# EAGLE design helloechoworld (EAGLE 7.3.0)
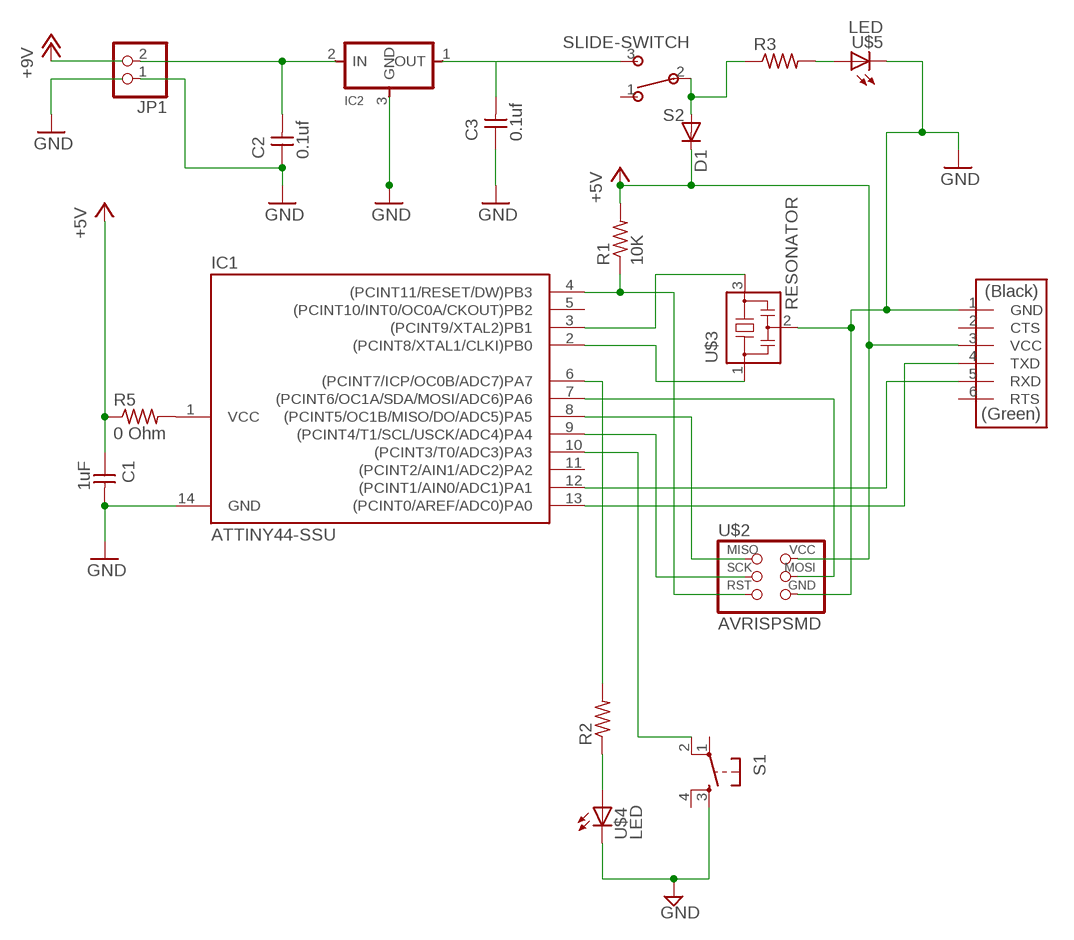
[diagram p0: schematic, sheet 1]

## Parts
C1  1uF  CAP-UNPOLARIZED  [C1206]
C2  0.1uf  CAP-UNPOLARIZED  [C1206]
C3  0.1uf  CAP-UNPOLARIZED  [C1206]
D1  DIODESOD123  [SOD123]
IC1  ATTINY44-SSU  [SOIC14]
IC2  REGULATORSOT23  [SOT23]
JP1  PINHD-1X2  [1X02]
R1  10K  RES-US1206  [R1206]
R2  RES-US1206  [R1206]
R3  RES-US1206  [R1206]
R5  0 Ohm  RES-US1206FAB  [R1206FAB]
S1  6MM_SWITCH6MM_SWITCH  [6MM_SWITCH]
S2  SLIDE-SWITCH  [AYZ0102AGRLC]
U$1  FTDI-SMD-HEADER  [1X06SMD]
U$2  AVRISPSMD  [2X03SMD]
U$3  RESONATOR  [EFOBM]
U$4  LED  [LED1206]
U$5  LED  [LED1206]

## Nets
+5V: C1.1 D1.CATHODE(C) R1.2 R5.1 U$1.3(VCC) U$2.2(VCC)
GND: C1.2 C2.1 C3.1 IC1.14(GND) IC2.3(GND) JP1.1 S1.3(S) U$1.1(GND) U$2.6(GND) U$3.2 U$4.2(C) U$5.2(C)
N$1: IC1.2((PCINT8/XTAL1/CLKI)PB0) U$3.1
N$2: IC1.8((PCINT5/OC1B/MISO/DO/ADC5)PA5) U$2.1(MISO)
N$3: IC1.3((PCINT9/XTAL2)PB1) U$3.3
N$4: IC1.6((PCINT7/ICP/OC0B/ADC7)PA7) R2.2
N$5: IC1.4((PCINT11/RESET/DW)PB3) R1.1 U$2.5(RST)
N$6: IC1.9((PCINT4/T1/SCL/USCK/ADC4)PA4) U$2.3(SCK)
N$7: IC1.7((PCINT6/OC1A/SDA/MOSI/ADC6)PA6) U$2.4(MOSI)
N$8: IC1.12((PCINT1/AIN0/ADC1)PA1) U$1.5(RXD)
N$9: IC1.13((PCINT0/AREF/ADC0)PA0) U$1.4(TXD)
N$10: R2.1 U$4.1(A)
N$11: IC1.10((PCINT3/T0/ADC3)PA3) S1.2(P1)
N$12: C2.2 IC2.2(IN) JP1.2
N$13: C3.2 IC2.1(OUT) S2.3
N$14: IC1.1(VCC) R5.2
N$16: D1.ANODE(A) R3.1 S2.2
N$17: R3.2 U$5.1(A)
Unconnected: IC1.5((PCINT10/INT0/OC0A/CKOUT)PB2) IC1.11((PCINT2/AIN1/ADC2)PA2) S1.1(P) S1.4(S1) S2.1 U$1.2(CTS) U$1.6(RTS)

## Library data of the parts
C1-C3 = fab:CAP-UNPOLARIZED
D1 = fab:DIODE: DIODE
IC1 = fab:ATTINY44
IC2 = fab:REGULATOR
JP1 = pinhead:PINHD-1X2: PIN HEADER
R1-R3 R5 = fab:RES-US: Resistor (US Symbol)
S1 = fab:6MM_SWITCH: OMRON SWITCH
S2 = fab:SLIDE-SWITCH: SMD slide-switch AYZ0102AGRLC as found in the fablab inventory. Includes the mounting holes. Made by Zaerc.
U$1 = fab:FTDI-SMD-HEADER
U$2 = fab:AVRISP
U$3 = fab:RESONATOR
U$4 U$5 = fab:LED: LED

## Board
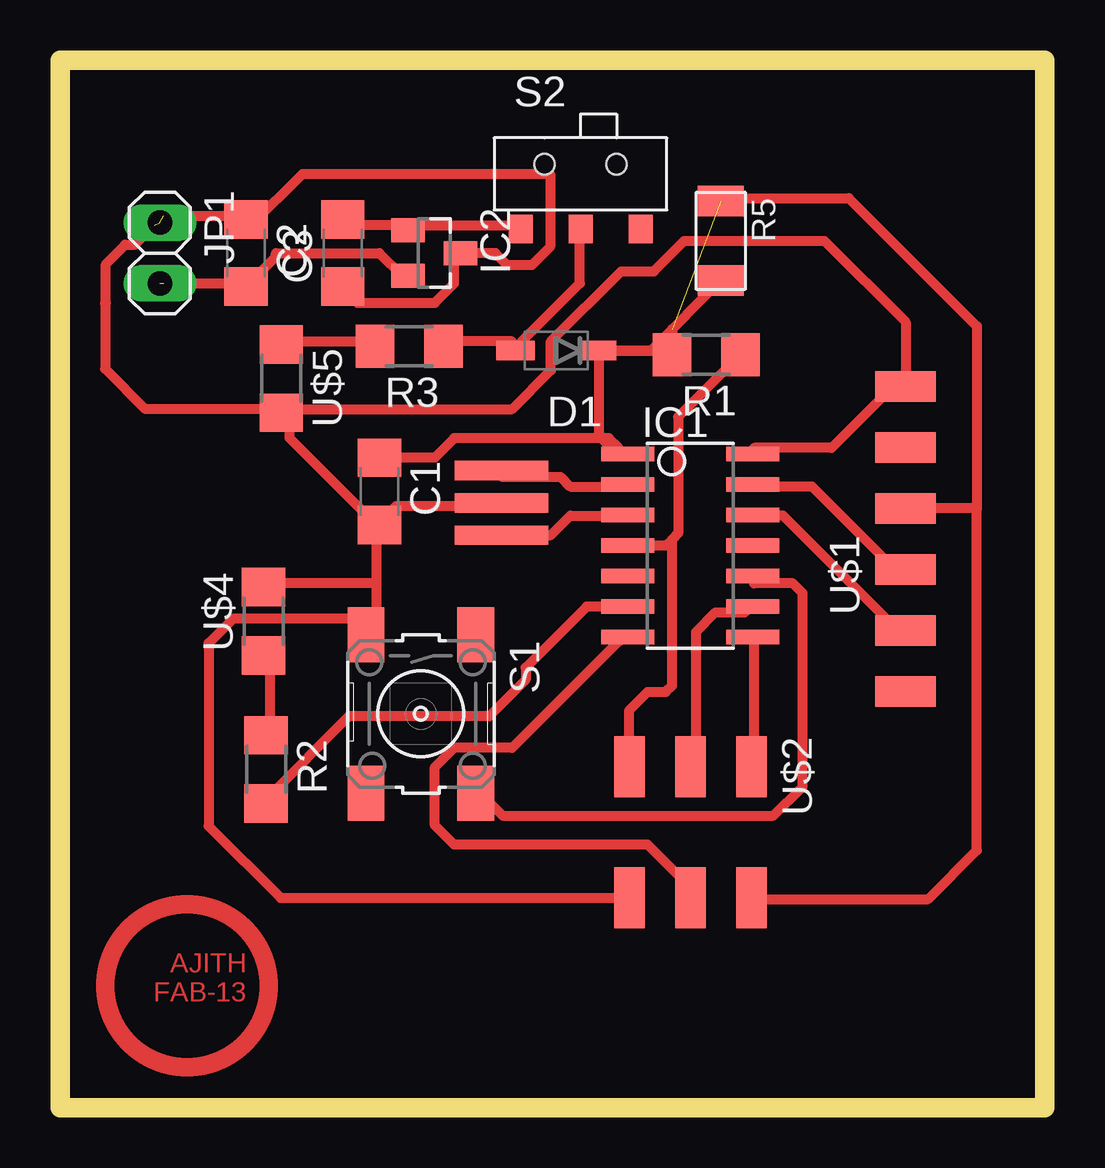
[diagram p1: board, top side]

Size 41.02 x 43.65 mm. Coordinates in mm from the lower left corner, seen from the top.
Outline: 0,0 41.02,0 41.02,43.65 0,43.65 0,0
Copper layers (1*16): Top 0.035mm / dielectric 1.5mm / Bottom 0.035mm
Design rules "default *": minimum track width 16mil, minimum drill 24mil, track to track 0.4mm, track to pad 0.4mm, pad to pad 0.4mm, via to via 0.4mm, smd to smd 0.4mm, copper to edge 40mil, drill to drill 16mil, minimum pad ring 10mil, minimum via ring 8mil, stop-mask expansion 4mil, vias tented up to drill 0mil, thermal gap 10mil

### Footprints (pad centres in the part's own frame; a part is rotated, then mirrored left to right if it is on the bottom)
C1206 = smd 1.6 x 1.8: 1 -1.4,0; 2 1.4,0
SOD123 = smd 1.6 x 0.8: ANODE 1.7,0; CATHODE -1.7,0
SOIC14 = smd 0.61 x 2.21: 1 -3.81,-2.603; 2 -2.54,-2.603; 3 -1.27,-2.603; 4 0,-2.603; 5 1.27,-2.603; 6 2.54,-2.603; 7 3.81,-2.603; 8 3.81,2.603; 9 2.54,2.603; 10 1.27,2.603; 11 0,2.603; 12 -1.27,2.603; 13 -2.54,2.603; 14 -3.81,2.603
SOT23 = smd 1 x 1.4: 1 -0.95,-1.1; 2 0.95,-1.1; 3 0,1.1
1X02 = drill 1.016 long: 1 -1.27,0; 2 1.27,0
R1206 = smd 1.6 x 1.803: 1 -1.422,0; 2 1.422,0
R1206FAB = smd 1.27 x 1.905: 1 -1.651,0; 2 1.651,0
6MM_SWITCH = smd 2.286 x 1.524: 1 -3.302,2.286; 2 3.302,2.286; 3 -3.302,-2.286; 4 3.302,-2.286
AYZ0102AGRLC = smd 1 x 1.2: 1 2.5,-2.3; 2 0,-2.3; 3 -2.5,-2.3 | hole 0.85: -1.5,0.4; 1.5,0.4
1X06SMD = smd 2.54 x 1.27: 1 0,6.35; 2 0,3.81; 3 0,1.27; 4 0,-1.27; 5 0,-3.81; 6 0,-6.35
2X03SMD = smd 2.54 x 1.27: 1 -2.54,2.54; 2 2.92,2.54; 3 -2.54,0; 4 2.92,0; 5 -2.54,-2.54; 6 2.92,-2.54
EFOBM = smd 0.8 x 3.9: 1 -1.35,0; 2 0,0; 3 1.35,0
LED1206 = smd 1.6 x 1.803: 1 -1.422,0; 2 1.422,0

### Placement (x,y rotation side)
C1  13.31,25.68 270 top
C2  7.75,35.61 270 top
C3  11.79,35.61 90 top
D1  20.68,31.55 180 top
IC1  26.26,23.42 270 top
IC2  15.6,35.61 270 top
JP1  4.17,35.61 270 top
R1  26.92,31.37 180 top
R2  8.59,14.1 270 top
R3  14.55,31.72 180 top
R5  27.53,36.12 270 top
S1  15.04,16.41 270 top
S2  21.69,38.91 0 top
U$1  35.23,23.7 0 top
U$2  26.26,11.66 270 top
U$3  18.39,25.2 270 top
U$4  8.48,20.27 90 top
U$5  9.22,30.38 270 top

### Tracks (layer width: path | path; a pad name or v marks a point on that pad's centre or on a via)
+5V  (1 unrouted)
  Top 0.406: 22.47,31.52 25.29,31.52 R1.2 25.5,32.44 | 22.47,27.89 22.87,27.89 23.28,27.49 | 22.47,27.89 16.42,27.89 15.62,27.09 13.6,27.09 C1.1 | 22.47,27.89 22.47,31.52 | 22.47,31.52 D1.CATHODE | R5.1 27.66,37.9 32.87,37.9 38.2,32.56 38.2,24.94 | 38.2,24.94 38.18,24.97 U$1.3 | U$2.2 28.86,8.69 36.17,8.69 38.2,10.72 38.2,24.94
GND  (2 unrouted)
  Top 0.406: 4.33,37.17 7.55,37.17 C2.1 7.96,36.76 10.11,38.91 20.42,38.91 20.42,35.86 19.66,35.1 18.64,35.1 18.14,35.61 IC2.3 16.42,35.55 16.42,34.34 15.62,33.54 12.39,33.54 11.99,33.94 C3.1 11.58,34.34 | IC1.14 28.92,27.49 32.15,27.49 34.97,30.31 U$1.1 35.23,32.74 31.85,36.12 26.01,36.12 24.74,34.85 23.38,34.85 20.46,31.92 20.46,30.71 18.84,29.1 9.57,29.1 U$5.2 | 13.2,21.84 13.2,20.23 12.79,19.83 S1.3 12.09,20.37 7.21,20.37 6.2,19.35 6.2,11.73 9.19,8.74 U$2.6 | 13.2,21.84 13.2,24.26 | 13.2,21.84 8.76,21.84 U$4.2 | 13.2,24.26 9.57,27.89 9.57,28.7 U$5.2 | 13.2,24.26 C1.2 13.6,24.67 14,25.07 18.04,25.07 U$3.2 | 3.92,36.76 3.12,35.96 2.71,35.96 1.91,35.15 1.91,33.54 1.88,33.51 1.88,30.78 3.56,29.1 9.17,29.1 U$5.2
N$1
  Top 0.406: IC1.2 23.28,25.88 21.26,25.88 20.86,26.28 18.44,26.28 U$3.1
N$2
  Top 0.406: IC1.8 28.92,19.43 28.92,14.59 U$2.1
N$3
  Top 0.406: IC1.3 23.28,24.67 21.26,24.67 20.46,23.86 18.44,23.86 U$3.3
N$4
  Top 0.406: IC1.6 21.95,20.88 19.41,18.34 19.41,17.83 17.88,16.31 12.04,16.31 8.59,12.85 R2.2
N$5
  Top 0.406: R1.1 25.76,28.78 25.76,23.93 25.5,23.67 | 25.5,23.67 25.25,23.42 IC1.4 | U$2.5 23.72,16.56 24.49,17.32 25.25,17.32 25.5,17.58 25.5,23.67
N$6
  Top 0.406: IC1.9 28.52,20.63 27.31,20.63 26.5,19.83 26.5,14.59 U$2.3
N$7
  Top 0.406: IC1.7 23.28,19.43 18.84,14.99 16.42,14.99 15.62,14.18 15.62,11.76 16.42,10.96 24.49,10.96 26.5,8.94 U$2.4
N$8
  Top 0.406: IC1.12 28.92,24.67 30.13,24.67 34.97,19.83 U$1.5
N$9
  Top 0.406: IC1.13 28.92,25.88 31.34,25.88 34.97,22.25 U$1.4
N$10
  Top 0.406: U$4.1 8.76,18.62 8.76,15.8 R2.1
N$11
  Top 0.406: IC1.10 28.92,21.84 30.54,21.84 30.94,21.44 30.94,13.38 29.73,12.17 18.44,12.17 17.63,12.97 S1.2
N$12  (1 unrouted)
  Top 0.406: 4.33,34.34 7.55,34.34 C2.2 8.99,35.46 8.99,35.61 13.31,35.61 14.26,34.66 IC2.2
N$13
  Top 0.406: S2.3 18.84,36.76 14.81,36.76 IC2.1 14.41,36.76 11.99,36.76 C3.2
N$14
  Top 0.406: R5.2 24.61,31.55 22.71,31.55 22.45,31.29 22.45,27.99 23.22,27.23 IC1.1
N$16
  Top 0.406: S2.2 21.66,36.36 21.66,34.34 19.25,31.92 D1.ANODE 18.84,31.92 16.02,31.92 R3.1
N$17
  Top 0.406: R3.2 12.79,31.92 9.57,31.92 U$5.1
(copper drawn outside any net)
  shapes: Top circle x1

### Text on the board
Top: AJITH / FAB-13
